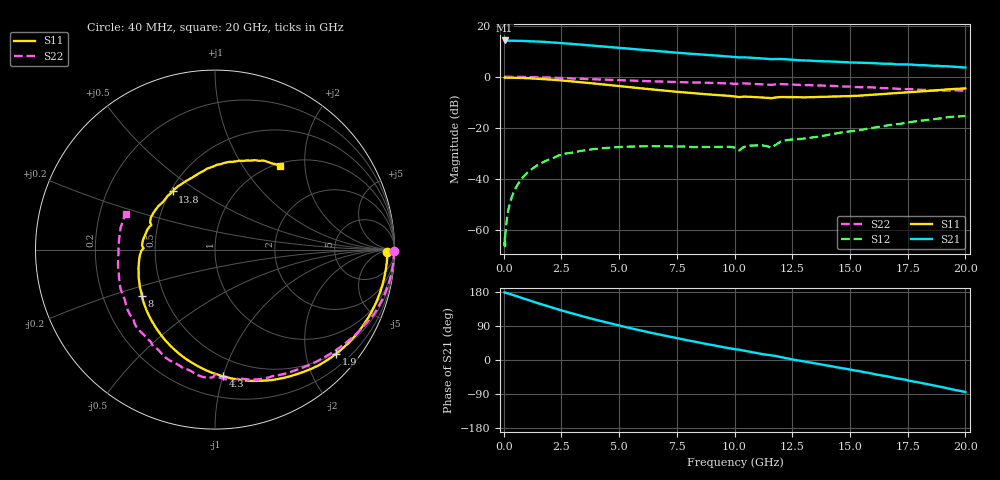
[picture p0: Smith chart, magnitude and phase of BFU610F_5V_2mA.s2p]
! Filename:  P:\Prog\Test\Noise\ATS_data\Testdata_Net\SplitFiles\BFU610_2W_A5_HighFreq_5V_2mA_D.s2p
! Date/Time: Wed 10/Aug/2011 16:58:10
! BFU610_2W_A5_HighFreq_5V_1mA_10mA_Bias2_R.s2p
! MDIF S-parameter v. bias file
! BFU610_2W_A5_HighFreq_5V_1mA_10mA
! Date/time Mon Aug 08 14:15:19 2011
! VAR V_out= 5.0010
! VAR I_out= 2.0100
! VAR V_in= 0.8591
! VAR I_in= 0.0137
! Device data file deembeded for feedlines and parallel
! Original file: \SplitFiles\BFU610_2W_A5_HighFreq_5V_2mA_R.s2p
! Feed-files: PR003V01_101208_Feed1.s2p, PR003V01_101208_Feed2.s2p
! Parallel-file: PR003V01_101208_Par.s2p
# MHz S MA R 50
!  Freq-MHz  S11-mag  S11-arg  S21-mag  S21-arg  S12-mag  S12-arg  S22-mag  S22-arg
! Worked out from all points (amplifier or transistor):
!   167 points, 40 MHz to 20 GHz, reference 50 ohm
!   highest |S21| = 14.2 dB at 40 MHz (marker M1)
!   |S21| within 3 dB of that: start of sweep to 5.115 GHz
!   unconditionally stable (mu >= 1): 6.999 GHz to 18.03 GHz
!   at 550 MHz: K = 0.02, MSG = 28.7 dB, |S12| = -43.2 dB
!   at 4.2 GHz: K = 0.49, MSG = 20.1 dB, |S12| = -28.1 dB
!   at 20 GHz: K = 0.85, MSG = 9.5 dB, |S12| = -15.4 dB
!   S11 on the Smith chart (normalised r, x): 40 MHz: 44, -15; 1.9 GHz: 0.47, -2.62; 4.3 GHz: 0.35, -1.00; 8 GHz: 0.37, -0.25; 13.8 GHz: 0.51, +0.40; 20 GHz: 1.05, +1.50
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40  0.9604 -0.8  5.154 178.2  0.0004719 71.5  0.996 -0.3
50  0.9551 -0.9  5.125 178.4  0.0006882 35.0  0.9967 -0.5
60  0.9631 -1.1  5.135 177.6  0.0004725 79.3  0.997 -0.5
80  0.9603 -1.7  5.132 177.6  0.0009115 82.6  0.9968 -0.8
180  0.9603 -3.9  5.093 176.0  0.002152 87.3  0.9969 -1.8
480  0.9548 -10.5  5.075 170.0  0.006024 85.7  0.9951 -4.9
1150  0.9313 -25.1  4.996 156.5  0.01456 75.5  0.9844 -11.8
1900  0.8899 -40.8  4.785 142.0  0.02309 64.7  0.9651 -19.2
2700  0.8299 -56.9  4.52 127.4  0.03109 53.5  0.9338 -26.6
3400  0.7769 -70.2  4.252 115.6  0.03529 46.0  0.909 -32.5
4300  0.7075 -86.4  3.937 101.3  0.03961 37.3  0.8775 -39.5
5400  0.6286 -105.3  3.563 85.2  0.0424 29.0  0.843 -47.7
6800  0.5417 -128.3  3.144 66.5  0.04318 21.7  0.8045 -57.4
8000  0.4823 -147.6  2.841 51.5  0.04244 18.1  0.7743 -65.5
9400  0.4322 -169.3  2.567 35.1  0.04194 20.0  0.7481 -75.4
10200  0.3981 178.9  2.391 27.2  0.03578 22.4  0.7256 -79.2
12000  0.3996 153.3  2.228 7.7  0.05327 39.5  0.7169 -93.2
13400  0.3989 131.3  2.047 -7.9  0.0647 32.9  0.677 -106.6
13800  0.4008 126.0  2.009 -12.0  0.06853 33.1  0.6672 -110.2
16800  0.4733 88.5  1.794 -45.5  0.1137 19.9  0.5916 -145.3
18400  0.5273 70.5  1.664 -64.7  0.143 6.6  0.548 -170.4
20000  0.5909 51.9  1.515 -84.6  0.17 -10.4  0.5367 158.2
